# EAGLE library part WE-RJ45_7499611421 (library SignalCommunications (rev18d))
Order Code 7499611421 Design THT xBase-T 10G Base-T Ports 1x1 Application Standard Tab Position UP LED (Left-Right) GREEN/YELLOW-GREEN EMI Fingers Yes Details see: http://katalog.we-online.de/en/pbs/WE-LAN_RJ45/7499611421? Updated by Yingchun Shan 2016-08-30 2016(C) Würth Elektronik
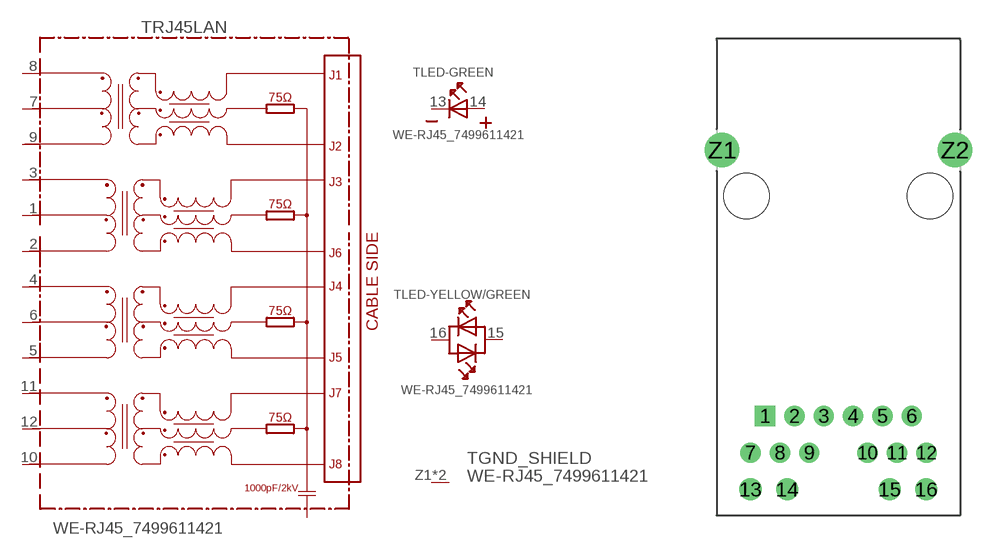
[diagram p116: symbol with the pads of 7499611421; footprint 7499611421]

Designator prefix T; gates RJ45LAN=7499611421 LED-GREEN=LED2PIN LED-YELLOW/GREEN=LED-DUAL-1 GND_SHIELD=GNDPIN

## WE-RJ45_7499611421 (COMPANY-URL: http://www.we-online.de; CREATED-BY: Christin Zierenner; CREATED-DATE: AUG 2012; DATASHEET-URL: http://katalog.we-online.de/kataloge/eisos/media/pdf/7499611421.pdf; MANUFACTURER: Würth Elektronik eiSos GmbH)  [7499611421]
1  RJ45LAN:1
2  RJ45LAN:2
3  RJ45LAN:3
4  RJ45LAN:4
5  RJ45LAN:5
6  RJ45LAN:6
7  RJ45LAN:7
8  RJ45LAN:8
9  RJ45LAN:9
10  RJ45LAN:10
11  RJ45LAN:11
12  RJ45LAN:12
13  LED-GREEN:K  pas
14  LED-GREEN:A  pas
15  LED-YELLOW/GREEN:AK2  pas
16  LED-YELLOW/GREEN:AK1  pas
Z1  GND_SHIELD:GND  pwr
Z2  GND_SHIELD:GND  pwr

## Footprint 7499611421 (pad centres in mm)
MAX HEIGHT=13.87mm PORTS----1X1 LED -YES
drill 0.9 square: 1 -5.075,-15.24
drill 0.9: 2 -3.045,-15.24; 3 -1.015,-15.24; 4 1.015,-15.24; 5 3.045,-15.24; 6 5.075,-15.24; 7 -6.095,-17.78; 8 -4.055,-17.78; 9 -2.025,-17.78; 10 2.025,-17.78; 11 4.055,-17.78; 12 6.095,-17.78
drill 1.02: 13 -6.09,-20.32; 14 -3.55,-20.32; 15 3.55,-20.32; 16 6.09,-20.32
drill 1.6: Z1 -8.065,3.18; Z2 8.065,3.18
hole 3.15 at -6.35,0
hole 3.15 at 6.35,0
